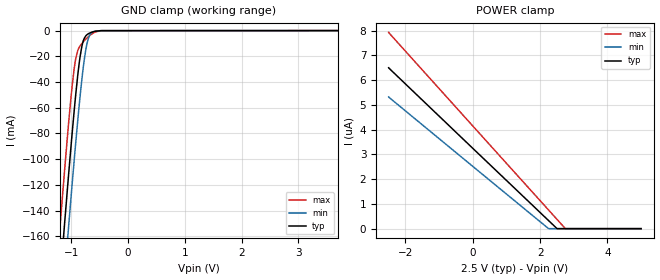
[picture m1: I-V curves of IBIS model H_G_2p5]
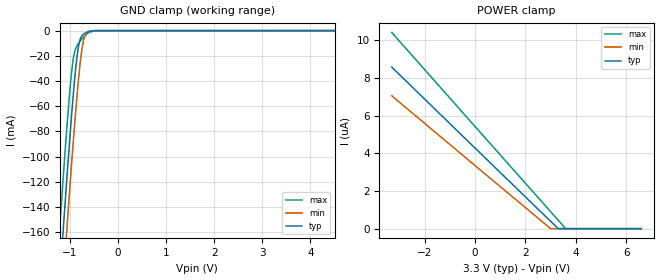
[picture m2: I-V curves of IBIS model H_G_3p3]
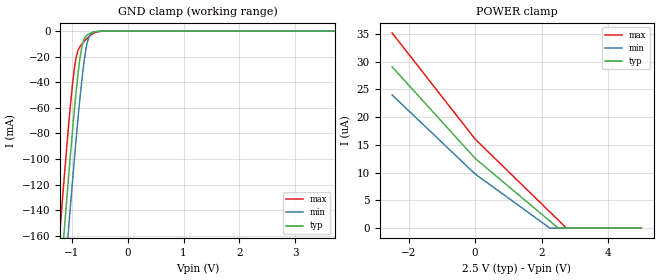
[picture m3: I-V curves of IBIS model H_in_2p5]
| Texas Instruments Incorporated
| 3.3V  LVCMOS High-Performance Clock Buffer
| Signal Rate: 200 kbps
| Marketing part#   Voltage Range   Package-type   #pins/pkg drawing
| cdclvc1112   2.25V - 3.6V   PW   24-pin TSSOP
[IBIS Ver]   4.1
[File name]   cdclvc1112.ibs
[File Rev]   1.0
[Date]   10/26/2010
[Source]   Model built from TISPICE simulations at:
   Texas Instruments Incorporated.
   Analog-eLab, HPA
   12500 TI Blvd
   Dallas, TX -75243
   For Support e-mail: elab_scm_ibis@list.ti.com
[Notes]   Revision History
   Rev 1.0: 07/09/2010
   - Model based on simulations from TIspiceD
   - C_comp values were obtained at 250MHz
   - For all buffers, Ccomp was obtained with the following corners:
   max C_comp was obtained at corner high VCC, low  temperature,
   strong process
   min C_comp was obtained at corner low  VCC, high temperature,
   weak process
   Rev 2.0: 08/03/2010
   Package information was updated
   Rev 2.0: 10/26/2010
   - Appl. Eng. requested corrections for Vinh & Vinl
   In H_in_2p5 Vinh should be 1.65V.
   In H_in_3p3 Vinl should be 1.05V.
[Disclaimer] This product is designed as an aid for customers of Texas
   Instruments.
   No warranties, either expressed or implied, with respect
   to this third party software (if any) or with respect to
   its fitness for any particular purpose is claimed by Texas
   Instruments or the author. The software (if any) is provided
   solely on an "as is" basis. The entire risk as to its quality
   and performance is with the customer
[Copyright]   (C)Copyright 2010 Texas Instruments Incorporated.
   All rights reserved.
|   Component cvclvc1112pw
[Component]   cdclvc1112
[Manufacturer]  Texas Instruments Incorporated
[Package]   |24-pin TSSOP package
|   typ   min   max
R_pkg   0.17344   0.07740   0.547663
L_pkg   3.33665nH   2.86513nH   3.98044nH
C_pkg   0.54766pF   0.44834pF   0.66133pF
[Pin] signal_name   model_name   R_pin   L_pin   C_pin
  1   CLKIN   H_in   0.16770  3.96810nH  0.66088pF
  2   1G   H_G   0.17620  3.66496nH  0.64292pF
  3   Y0   H_out   0.19494  3.49539nH  0.55063pF
  4   GND   GND   0.19042  3.21906nH  0.49011pF
  5   VDD   POWER   0.18491  3.05344nH  0.48225pF
  6   Y4   H_out   0.17369  2.89213nH  0.45163pF
  7   GND   GND   0.17097  2.86513nH  0.44876pF
  8   Y6   H_out   0.17490  2.95523nH  0.47744pF
  9   VDD   POWER   0.18207  3.13880nH  0.48756pF
 10   Y9   H_out   0.18253  3.37611nH  0.54440pF
 11   GND   GND   0.17626  3.67358nH  0.64390pF
 12   Y11   H_out   0.16786  3.98044nH  0.66085pF
 13   VDD   POWER   0.16785  3.97630nH  0.66133pF
 14   Y10   H_out   0.17644  3.67337nH  0.64485pF
 15   GND   GND   0.18250  3.37509nH  0.54507pF
 16   Y8   H_out   0.18156  3.13356nH  0.48686pF
 17   Y7   H_out   0.17490  2.95523nH  0.47681pF
 18   VDD   POWER   0.17098  2.86573nH  0.44834pF
 19   Y5   H_out   0.17366  2.89093nH  0.44974pF
 20   GND   GND   0.17992  3.00322nH  0.48004pF
 21   Y2   H_out   0.19041  3.21900nH  0.49539pF
 22   VDD   POWER   0.07740  3.05958nH  0.60735pF
 23   Y3   H_out   0.17650  3.66989nH  0.64602pF
 24   Y1   H_out   0.16802  3.97543nH  0.66079pF
[Pin Mapping]pulldown_ref pullup_ref gnd_clamp_ref power_clamp_ref |ext_ref
 1   NC   NC   GNDBUS   PWRBUS   | CLKIN
 2   NC   NC   GNDBUS   PWRBUS   | 1G
 3   GNDBUS   PWRBUS   NC   NC   | Y0
 4   GNDBUS   NC   | GND
 5   NC   PWRBUS   | VDD
 6   GNDBUS   PWRBUS   NC   NC   | Y4
 7   GNDBUS   NC   | GND
 8   GNDBUS   PWRBUS   NC   NC   | Y6
 9   NC   PWRBUS   | VDD
10   GNDBUS   PWRBUS   NC   NC   | Y9
11   GNDBUS   NC   | GND
12   GNDBUS   PWRBUS   NC   NC   | Y11
13   NC   PWRBUS   | VDD
14   GNDBUS   PWRBUS   NC   NC   | Y10
15   GNDBUS   NC   | GND
16   GNDBUS   PWRBUS   NC   NC   | Y8
17   GNDBUS   PWRBUS   NC   NC   | Y7
18   NC   PWRBUS   | VDD
19   GNDBUS   PWRBUS   NC   NC   | Y5
20   GNDBUS   NC   | GND
21   GNDBUS   PWRBUS   NC   NC   | Y2
22   NC   PWRBUS   | VDD
23   GNDBUS   PWRBUS   NC   NC   | Y3
24   GNDBUS   PWRBUS   NC   NC   | Y1
[Model Selector] H_G
H_G_2p5   H_G Input model  at 2.5V
H_G_3p3   H_G Input model  at 3.3V
[Model Selector] H_in
H_in_2p5   H_in Input model at 2.5V
H_in_3p3   H_in Input model at 3.3V
[Model Selector] H_out
H_out_2p5   H_out Output model at 2.5V
H_out_3p3   H_out Output model at 3.3V
| Models and submodels in the file (6): H_G_2p5 (Input), H_G_3p3 (Input), H_in_2p5 (Input), H_in_3p3 (Input), H_out_2p5 (Output), H_out_3p3 (Output)
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|   H_G_2p5
[Model]   H_G_2p5
|Signal:   1G
Model_type   Input
Vinl   = 0.85
Vinh   = 1.65
|   typ   min   max
C_comp   910fF   809fF   967fF
[Voltage Range]   2.5   2.25   2.75
[Temperature Range]   25   85   -40
[Power Clamp Reference]   2.5   2.25   2.75
[GND Clamp Reference]   0   0   0
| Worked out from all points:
|   GND clamp passes 1 mA (typ) near -0.62 V on its own axis
[GND Clamp]
|   Voltage   I(typ)   I(min)   I(max)
-2.5V     -968.1mA   -1.007A    -929mA
-1.21V    -199mA     -240.4mA   -156.9mA
-1.15V    -165.5mA   -206.8mA   -123.9mA
-1.12V    -149.1mA   -190.2mA   -107.7mA
-1.064V   -118.8mA   -159.4mA   -78.45mA
-1.045V   -108.9mA   -149.3mA   -69.13mA
-947.5mV  -60.05mA   -98.34mA   -28.07mA
-850mV    -20.81mA   -51.87mA   -12.03mA
-771.2mV  -5.755mA   -21.65mA   -7.739mA
-681.3mV  -1.974mA   -3.841mA   -3.953mA
-463.7mV  -54uA      -32.29uA   -94.42uA
5V        0A         0A         0A
[POWER Clamp]
|   Voltage   I(typ)   I(min)   I(max)
-2.5V     6.5uA      5.321uA    7.929uA
2.251V    325.7nA    0A         752.1nA
2.502V    0A         0A         373.2nA
2.75V     0A         0A         0A
5V        0A         0A         0A
|   H_G_3p3
[Model]   H_G_3p3
|Signal:   1G
Model_type   Input
Vinl   = 1.05
Vinh   = 2.25
|   typ   min   max
C_comp   831.2f   785f   940.5f
[Voltage Range]   3.3   3   3.6
[Temperature Range]   25   85   -40
[Power Clamp Reference]   3.3   3   3.6
[GND Clamp Reference]   0   0   0
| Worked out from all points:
|   GND clamp passes 1 mA (typ) near -0.62 V on its own axis
[GND Clamp]
|   Voltage   I(typ)   I(min)   I(max)
-3.3V     -1.461A    -1.498A    -1.424A
-1.221V   -205.1mA   -246.6mA   -163.1mA
-1.206V   -196.8mA   -238.2mA   -154.8mA
-1.137V   -158.3mA   -199.5mA   -116.7mA
-1.063V   -118.2mA   -158.8mA   -77.87mA
-993.3mV  -82.31mA   -121.9mA   -45.27mA
-933.9mV  -53.76mA   -91.51mA   -24.11mA
-834.9mV  -16.5mA    -45.37mA   -11.07mA
-790.3mV  -7.806mA   -28.02mA   -8.666mA
-730.9mV  -3.374mA   -11.05mA   -5.922mA
-632mV    -1.127mA   -1.236mA   -2.355mA
6.6V      0A         0A         0A
[POWER Clamp]
|   Voltage   I(typ)   I(min)   I(max)
-3.3V     8.58uA     7.058uA    10.42uA
3.001V    391.5nA    0A         903.2nA
3.303V    0A         0A         447.8nA
3.6V      0A         0A         0A
6.6V      0A         0A         0A
|   H_in_2p5
[Model]   H_in_2p5
|Signal:   CLK_IN
Model_type   Input
Vinl   = 0.85
Vinh   = 1.65
|   typ   min   max
C_comp   0.943pF   0.765pF   1.207pF
[Voltage Range]   2.5   2.25   2.75
[Temperature Range]   25   85   -40
[Power Clamp Reference]   2.5   2.25   2.75
[GND Clamp Reference]   0   0   0
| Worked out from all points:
|   GND clamp passes 1 mA (typ) near -0.62 V on its own axis
[GND Clamp]
|   Voltage   I(typ)   I(min)   I(max)
-2.5V     -968.1mA   -1.007A    -929mA
-1.21V    -199mA     -240.4mA   -156.9mA
-1.15V    -165.6mA   -206.8mA   -123.9mA
-1.12V    -149.1mA   -190.2mA   -107.7mA
-1.064V   -118.8mA   -159.4mA   -78.47mA
-1.045V   -108.9mA   -149.3mA   -69.14mA
-947.5mV  -60.06mA   -98.34mA   -28.08mA
-850mV    -20.82mA   -51.87mA   -12.04mA
-771.2mV  -5.763mA   -21.66mA   -7.749mA
-681.3mV  -1.981mA   -3.847mA   -3.963mA
-463.7mV  -60.38uA   -37.46uA   -102.3uA
5V        0A         0A         0A
[POWER Clamp]
|   Voltage   I(typ)   I(min)   I(max)
-2.5V     29.05uA    23.98uA    35.15uA
1.25mV    12.55uA    9.742uA    16.01uA
2.251V    1.261uA    0A         2.905uA
2.502V    0A         0A         1.442uA
2.75V     0A         0A         0A
5V        0A         0A         0A
